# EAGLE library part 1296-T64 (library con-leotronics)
1.27mm SINGLE ROW FEMALE SOCKET Source: http://www.leotronics.co.uk/Conexcon/Data%20Sheets/sec.%20A/1296ing.pdf
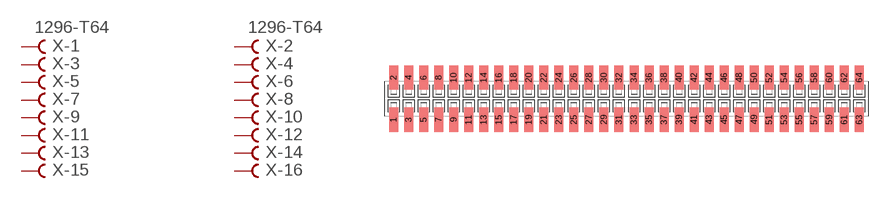
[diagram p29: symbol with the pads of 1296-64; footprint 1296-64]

Designator prefix X; gates -1=FVAL -2=FVAL -3=F -4=F -5=F -6=F -7=F -8=F -9=F -10=F -11=F -12=F -13=F -14=F -15=F -16=F -17=F -18=F -19=F -20=F -21=F -22=F -23=F -24=F -25=F -26=F -27=F -28=F -29=F -30=F -31=F -32=F -33=F -34=F -35=F -36=F -37=F -38=F -39=F -40=F -41=F -42=F -43=F -44=F -45=F -46=F -47=F -48=F -49=F -50=F -51=F -52=F -53=F -54=F -55=F -56=F -57=F -58=F -59=F -60=F -61=F -62=F -63=F -64=F

## 1296-T64 (OC_FARNELL: unknown; OC_NEWARK: unknown)  [1296-64]
1  -1:B  pas
2  -2:B  pas
3  -3:B  pas
4  -4:B  pas
5  -5:B  pas
6  -6:B  pas
7  -7:B  pas
8  -8:B  pas
9  -9:B  pas
10  -10:B  pas
11  -11:B  pas
12  -12:B  pas
13  -13:B  pas
14  -14:B  pas
15  -15:B  pas
16  -16:B  pas
17  -17:B  pas
18  -18:B  pas
19  -19:B  pas
20  -20:B  pas
21  -21:B  pas
22  -22:B  pas
23  -23:B  pas
24  -24:B  pas
25  -25:B  pas
26  -26:B  pas
27  -27:B  pas
28  -28:B  pas
29  -29:B  pas
30  -30:B  pas
31  -31:B  pas
32  -32:B  pas
33  -33:B  pas
34  -34:B  pas
35  -35:B  pas
36  -36:B  pas
37  -37:B  pas
38  -38:B  pas
39  -39:B  pas
40  -40:B  pas
41  -41:B  pas
42  -42:B  pas
43  -43:B  pas
44  -44:B  pas
45  -45:B  pas
46  -46:B  pas
47  -47:B  pas
48  -48:B  pas
49  -49:B  pas
50  -50:B  pas
51  -51:B  pas
52  -52:B  pas
53  -53:B  pas
54  -54:B  pas
55  -55:B  pas
56  -56:B  pas
57  -57:B  pas
58  -58:B  pas
59  -59:B  pas
60  -60:B  pas
61  -61:B  pas
62  -62:B  pas
63  -63:B  pas
64  -64:B  pas

## Footprint 1296-64 (pad centres in mm)
1.27mm SINGLE ROW FEMALE SOCKET Source: http://www.leotronics.co.uk/Conexcon/Data%20Sheets/sec.%20A/1296ing.pdf
smd 0.76 x 2.05: 1 -19.685,-1.78; 2 -19.685,1.78; 3 -18.415,-1.78; 4 -18.415,1.78; 5 -17.145,-1.78; 6 -17.145,1.78; 7 -15.875,-1.78; 8 -15.875,1.78; 9 -14.605,-1.78; 10 -14.605,1.78; 11 -13.335,-1.78; 12 -13.335,1.78; 13 -12.065,-1.78; 14 -12.065,1.78; 15 -10.795,-1.78; 16 -10.795,1.78; 17 -9.525,-1.78; 18 -9.525,1.78; 19 -8.255,-1.78; 20 -8.255,1.78; 21 -6.985,-1.78; 22 -6.985,1.78; 23 -5.715,-1.78; 24 -5.715,1.78; 25 -4.445,-1.78; 26 -4.445,1.78; 27 -3.175,-1.78; 28 -3.175,1.78; 29 -1.905,-1.78; 30 -1.905,1.78; 31 -0.635,-1.78; 32 -0.635,1.78; 33 0.635,-1.78; 34 0.635,1.78; 35 1.905,-1.78; 36 1.905,1.78; 37 3.175,-1.78; 38 3.175,1.78; 39 4.445,-1.78; 40 4.445,1.78; 41 5.715,-1.78; 42 5.715,1.78; 43 6.985,-1.78; 44 6.985,1.78; 45 8.255,-1.78; 46 8.255,1.78; 47 9.525,-1.78; 48 9.525,1.78; 49 10.795,-1.78; 50 10.795,1.78; 51 12.065,-1.78; 52 12.065,1.78; 53 13.335,-1.78; 54 13.335,1.78; 55 14.605,-1.78; 56 14.605,1.78; 57 15.875,-1.78; 58 15.875,1.78; 59 17.145,-1.78; 60 17.145,1.78; 61 18.415,-1.78; 62 18.415,1.78; 63 19.685,-1.78; 64 19.685,1.78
